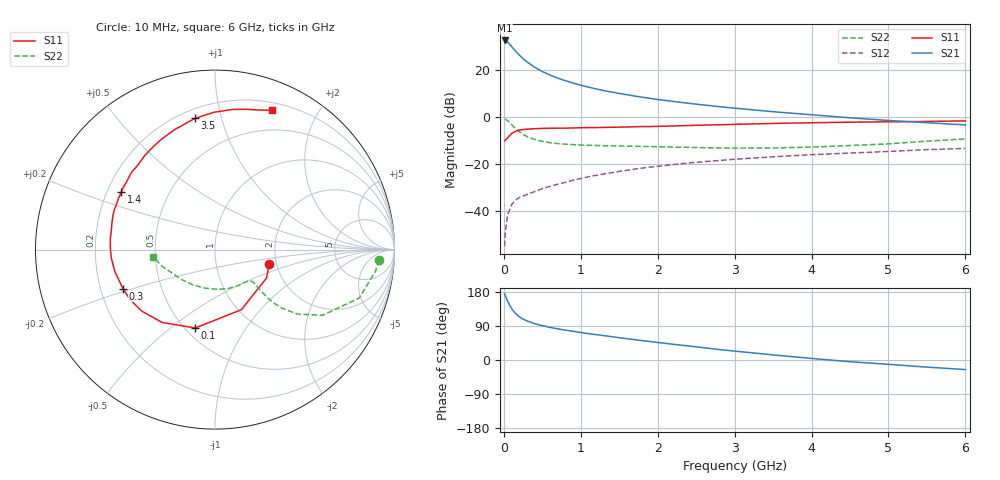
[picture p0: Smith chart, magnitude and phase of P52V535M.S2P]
! SIEMENS Small Signal Semiconductors
! BFP183
! Si NPN RF Bipolar Junction Transistor in SOT143
! VCE = 2.5 V  IC = 35 mA
! Common Emitter S-Parameters:  March  1996
# GHz  S  MA  R  50
!  f  S11  S21  S12  S22
! GHz  MAG  ANG  MAG  ANG  MAG  ANG  MAG  ANG
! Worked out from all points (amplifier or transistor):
!   36 points, 10 MHz to 6 GHz, reference 50 ohm
!   highest |S21| = 32.7 dB at 10 MHz (marker M1)
!   |S21| within 3 dB of that: start of sweep to 112 MHz
!   unconditionally stable (mu >= 1): 473 MHz to 5.904 GHz
!   at 250 MHz: K = 0.71, MSG = 29.2 dB, |S12| = -33.6 dB
!   at 1.4 GHz: K = 1.26, MAG = 14.1 dB, |S12| = -23.6 dB
!   at 6 GHz: K = 0.99, MSG = 5.0 dB, |S12| = -13.3 dB
!   S11 on the Smith chart (normalised r, x): 10 MHz: 1.83, -0.33; 100 MHz: 0.56, -0.61; 300 MHz: 0.30, -0.19; 1.4 GHz: 0.26, +0.27; 3.5 GHz: 0.26, +0.83; 6 GHz: 0.28, +1.45
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0.01  0.3136 -14.9  43.26 174.7  0.0018 81.6  0.915 -3.6
0.02  0.3279 -29.1  42.89 169.7  0.0036 83.8  0.9022 -7.7
0.05  0.3656 -66.3  39.98 154.6  0.0086 73.1  0.8472 -18.6
0.1  0.4503 -104.1  32.25 135.9  0.0137 59.0  0.7024 -31.4
0.15  0.5018 -126.0  25.97 123.1  0.0172 53.4  0.5818 -38.1
0.2  0.534 -140.3  21.25 114.3  0.0196 51.6  0.4953 -41.2
0.25  0.5491 -149.9  17.67 107.9  0.021 50.4  0.4347 -42.4
0.3  0.5571 -157.1  15.14 103.3  0.0228 50.7  0.3905 -42.5
0.4  0.5714 -167.7  11.7 95.9  0.0261 53.7  0.3377 -41.8
0.5  0.5791 -174.9  9.418 90.6  0.0302 54.2  0.3069 -41.2
0.6  0.583 179.4  7.96 86.1  0.0339 56.1  0.288 -40.6
0.7  0.5863 174.1  6.799 82.3  0.0377 57.7  0.2753 -40.6
0.8  0.5872 169.9  6.018 78.8  0.0412 58.3  0.2677 -40.9
1.1  0.6033 158.1  4.392 69.6  0.0542 59.0  0.2529 -43.6
1.4  0.6124 148.3  3.453 61.7  0.0662 57.9  0.2462 -48.1
1.8  0.6342 136.8  2.677 51.1  0.0828 55.8  0.2387 -56.0
2.2  0.6547 126.6  2.178 41.5  0.0984 52.2  0.2319 -65.4
2.8  0.6932 112.2  1.684 27.6  0.1202 46.5  0.2232 -82.2
3.5  0.7397 98.7  1.315 13.4  0.1442 39.9  0.2221 -104.7
4.5  0.7863 83.1  0.975 -4.5  0.1735 30.4  0.2498 -138.0
5.5  0.8155 72.5  0.766 -18.8  0.2047 21.9  0.3102 -162.7
6  0.8382 67.8  0.687 -25.3  0.2175 17.0  0.3469 -173.2
